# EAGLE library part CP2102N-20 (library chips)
A cheap, simple USB to UART adapter
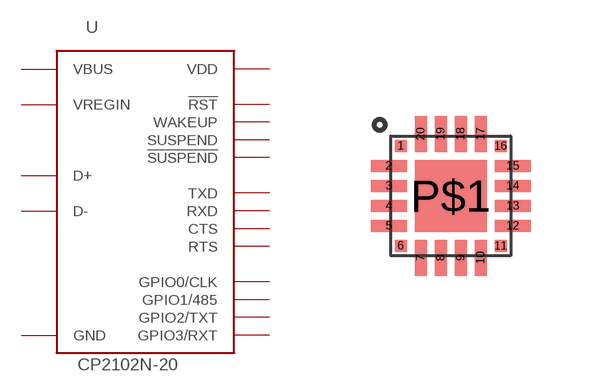
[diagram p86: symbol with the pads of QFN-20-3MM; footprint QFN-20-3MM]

Designator prefix U

## CP2102N-20 (DIGIKEY: 336-3692-ND; MANUFACTURER: SiLabs; MPN: CP2102N-A01-GQFN20)  [QFN-20-3MM]
1  GPIO1/485
2  GPIO0/CLK
3  GND
4  D+
5  D-
6  VDD
7  VREGIN
8  VBUS
9  !RST
11  !SUSPEND
12  GND
13  WAKEUP
14  SUSPEND
15  CTS
16  RTS
17  RXD
18  TXD
19  GPIO3/RXT
20  GPIO2/TXT
P$1  GND

## Footprint QFN-20-3MM (pad centres in mm)
smd 0.3 x 0.3: 1 -1.25,1.25; 6 -1.25,-1.25; 11 1.25,-1.25; 16 1.25,1.25
smd 0.9 x 0.3: 2 -1.55,0.75; 3 -1.55,0.25; 4 -1.55,-0.25; 5 -1.55,-0.75; 12 1.55,-0.75; 13 1.55,-0.25; 14 1.55,0.25; 15 1.55,0.75
smd 0.3 x 0.9: 7 -0.75,-1.55; 8 -0.25,-1.55; 9 0.25,-1.55; 10 0.75,-1.55; 17 0.75,1.55; 18 0.25,1.55; 19 -0.25,1.55; 20 -0.75,1.55
smd 1.8 x 1.8: P$1 0,0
